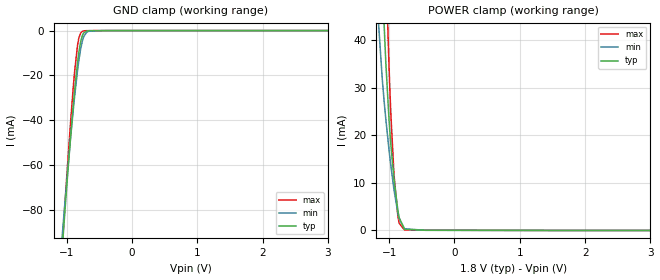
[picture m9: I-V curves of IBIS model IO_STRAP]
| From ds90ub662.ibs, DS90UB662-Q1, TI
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|   IO_STRAP Model
[Model]   IO_STRAP
Model_type   Input
Vinl = 0.54
Vinh = 1.26
|   typ   min   max
C_comp   0.310pF   0.249pF   0.402pF
[Voltage Range]   1.8   1.71   1.89
[Temperature Range]   27   105   -40
[Power Clamp Reference]   1.8   1.71   1.89
[GND Clamp Reference]   0   0   0
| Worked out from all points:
|   GND clamp passes 1 mA (typ) near -0.74 V on its own axis
|   POWER clamp passes 1 mA (typ) near -0.79 V on its own axis
[GND Clamp]
|   Voltage   I(typ)   I(min)   I(max)
-1.8V     -431.7mA   -399.8mA   -451.7mA
-1.157V   -136.1mA   -125.5mA   -138.1mA
-1.055V   -92.5mA    -87.21mA   -90.67mA
-1.012V   -75.04mA   -72.04mA   -71.4mA
-936mV    -46.52mA   -47.07mA   -39.68mA
-876.6mV  -26.7mA    -29.31mA   -18.23mA
-833.4mV  -14.56mA   -18.05mA   -6.777mA
-811.8mV  -9.629mA   -13.23mA   -3.267mA
-757.8mV  -2.152mA   -4.557mA   -320uA
-666mV    -79.2uA    -329.9uA   -20.56uA
-444.6mV  -9.322uA   -8.25uA    -11.12uA
3.6V      0A         0A         0A
[POWER Clamp]
|   Voltage   I(typ)   I(min)   I(max)
-1.8V     450.2mA    350.1mA    527.5mA
-1.174V   83.68mA    46.04mA    124.1mA
-1.076V   43.49mA    27.25mA    69.61mA
-1.071V   41.71mA    26.43mA    66.81mA
-1.049V   35.09mA    23.3mA     55.99mA
-1.001V   23.25mA    16.92mA    34.42mA
-973.8mV  18.15mA    13.72mA    24.65mA
-925.2mV  10.78mA    8.553mA    11.76mA
-865.8mV  4.239mA    3.681mA    3.051mA
-844.2mV  2.625mA    2.445mA    1.501mA
-763.2mV  243uA      346.7uA    107.6uA
3.6V      0A         0A         0A
